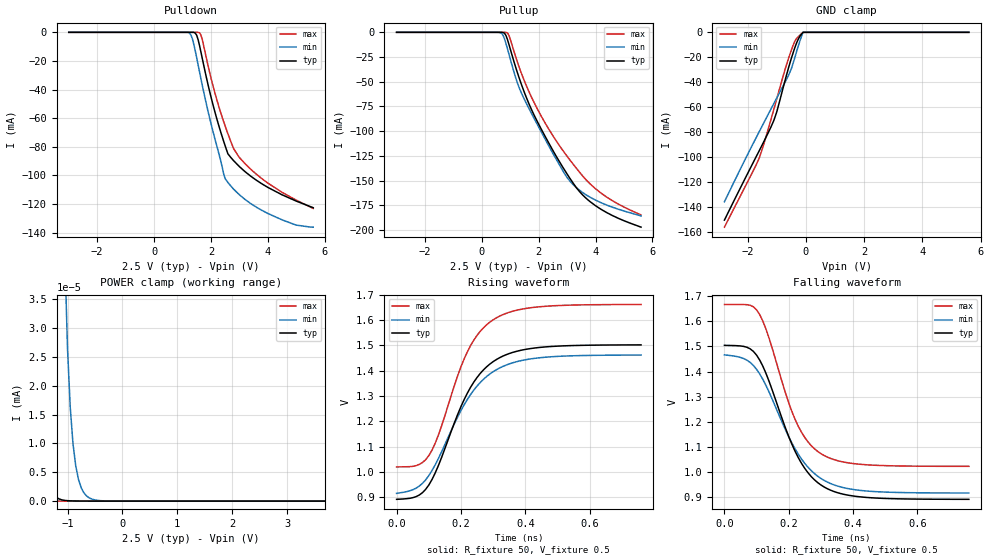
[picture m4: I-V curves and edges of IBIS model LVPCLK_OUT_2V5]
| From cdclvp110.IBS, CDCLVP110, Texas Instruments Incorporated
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|   Diff. Driver Output Model for 2.5V VCC range   |
[Model]   LVPCLK_OUT_2V5
Model_type   3-state_ECL
| Signals   Y0,Y0-, Y1,Y1-, y2,Y2-, y3,y3-, y4,y4-
|   y5,y5-, y6,y6-, y7,y7-, y8,y8-, y9,y9-
| variable   typ   min   max
C_comp   2.5pF   NA   NA
Cref = 0pF   |load capacitance for timing spec
Rref = 50   |50 to VCC-2
Vref = 0.5   |Timing specification test load voltage, VCC-2V
Vmeas = 1.19V   |Vref for timing measurements (x-point)
[Model Spec]
Vmeas   1.19V   1.19V   1.34V
| Vmeas is the expected cross point for each differential signal pair.
|Vref   0.5V   0.375V   0.75V
[Temperature Range]   40C   110C   -40C
[Voltage range]   2.5V   2.375V   2.75V
[Pulldown reference]   2.5V   2.375V   2.75V
[GND Clamp reference]   0V   0V   0V
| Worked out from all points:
|   GND clamp passes 1 mA (typ) near -0.13 V on its own axis
|   POWER clamp passes 1 mA (typ) near -2.41 V on its own axis
|   rising waveform, R_fixture 50, V_fixture 0.5: 20-80 % time 128ps typ, 141ps min, 116ps max; typ from 0.892 V to 1.5 V
|   falling waveform, R_fixture 50, V_fixture 0.5: 20-80 % time 118ps typ, 130ps min, 106ps max; typ from 1.5 V to 0.893 V
[Pullup]
|   40C:2.5V:nominal  110C:2.375V:weak  -40C:2.75V:strong
|  Voltage   I(typ)   I(min)   I(max)
-3V       43.55pA    161.8pA    42.73pA
600mV     -1.061uA   -79.39uA   -394.3pA
800mV     -1.024mA   -6.921mA   -6.028uA
950mV     -12mA      -21.81mA   -2.901mA
1.2V      -36.29mA   -46.84mA   -25.72mA
1.4V      -53.39mA   -61.94mA   -42.17mA
1.7V      -75.17mA   -79.47mA   -62.77mA
2.1V      -98.52mA   -101.3mA   -85.41mA
3V        -143.4mA   -147mA     -125.5mA
3.45V     -161.6mA   -160.1mA   -142mA
4V        -175.5mA   -169.8mA   -158.3mA
5.6V      -197.1mA   -185.7mA   -184.8mA
[Pulldown]
|   40C:2.5V:nominal  110C:2.375V:weak  -40C:2.75V:strong
|  Voltage   I(typ)   I(min)   I(max)
-3V       4.257fA    103.4fA    42.69pA
1.25V     -128nA     -620.5uA   -23.55pA
1.35V     -3.831uA   -4.537mA   -1.087nA
1.5V      -2.018mA   -17.72mA   -1.137uA
1.65V     -13.77mA   -32.5mA    -1.862mA
2.05V     -48.79mA   -67.44mA   -35.55mA
2.5V      -79.2mA    -102.2mA   -65.37mA
2.6V      -84.98mA   -105mA     -70.96mA
2.8V      -89.73mA   -109.6mA   -81.35mA
3.4V      -100.5mA   -119.7mA   -95.68mA
4.5V      -113.6mA   -131.1mA   -111.8mA
5.6V      -122.6mA   -136.2mA   -123.1mA
[POWER Clamp]
|   40C:2.5V:nominal  110C:2.375V:weak  -40C:2.75V:strong
|  Voltage   I(typ)   I(min)   I(max)
-3V       20.03mA    31.02mA    4.131mA
-2.1V     28.57uA    976.7uA    36.79nA
-2.05V    15.82uA    637.9uA    16.46nA
-2V       8.748uA    409uA      7.373nA
-1.8V     809.9nA    62.77uA    315.9pA
-1.55V    40.93nA    5.618uA    22.82pA
-1.4V     6.824nA    1.308uA    14.81pA
-1.15V    365.7pA    114.5nA    9.648pA
-1.05V    125.7pA    43.14nA    8.021pA
-850mV    26.98pA    6.121nA    5.224pA
-600mV    11.8pA     540.8pA    2.571pA
5.6V      0A         0A         0A
[GND Clamp]
|   40C:2.5V:nominal  110C:2.375V:weak  -40C:2.75V:strong
|  Voltage   I(typ)   I(min)   I(max)
-2.8V     -150.5mA   -135.8mA   -156.2mA
-1.6V     -94.71mA   -79.41mA   -100.5mA
-1.4V     -85.42mA   -70.4mA    -85.86mA
-1.1V     -70.49mA   -56.97mA   -61.55mA
-1V       -63.63mA   -52.52mA   -53.16mA
-700mV    -37.1mA    -39.23mA   -28.45mA
-500mV    -20.78mA   -29.16mA   -14.15mA
-400mV    -13.59mA   -21.8mA    -8.095mA
-300mV    -7.377mA   -13.83mA   -4.322mA
-200mV    -2.996mA   -6.46mA    -2.121mA
-100mV    0A         0A         0A
5.6V      0A         0A         0A
[ramp]
| variable   typ   min   max
dV/dt_r   0.3382/1.1442E-10   0.2939/1.2180E-10   0.3561/1.0430E-10
dV/dt_f   0.3382/1.0704E-10   0.2939/1.1394E-10   0.3561/9.6031E-11
[Rising Waveform]
R_fixture = 50
V_fixture = 0.5
V_fixture_min = 0.375
V_fixture_max = 0.75
|   40C:2.5V:nominal  110C:2.375V:weak  -40C:2.75V:strong
|  Voltage   I(typ)   I(min)   I(max)
0s        892.3mV    915.8mV    1.02V
60ps      902.6mV    935.9mV    1.025V
100ps     948.5mV    985.7mV    1.065V
130ps     1.026V     1.054V     1.146V
190ps     1.228V     1.218V     1.381V
220ps     1.312V     1.287V     1.475V
260ps     1.389V     1.354V     1.556V
300ps     1.436V     1.396V     1.601V
440ps     1.492V     1.451V     1.652V
760ps     1.502V     1.462V     1.662V
[Falling Waveform]
R_fixture = 50
V_fixture = 0.5
V_fixture_min = 0.375
V_fixture_max = 0.75
|   40C:2.5V:nominal  110C:2.375V:weak  -40C:2.75V:strong
|  Voltage   I(typ)   I(min)   I(max)
0s        1.504V     1.467V     1.667V
70ps      1.497V     1.446V     1.666V
110ps     1.445V     1.39V      1.626V
130ps     1.391V     1.343V     1.566V
190ps     1.175V     1.168V     1.314V
220ps     1.083V     1.093V     1.21V
260ps     998mV      1.02V      1.121V
300ps     949.7mV    975.6mV    1.074V
430ps     901.6mV    927.2mV    1.031V
760ps     892.7mV    917.8mV    1.024V
